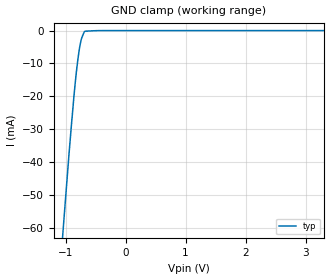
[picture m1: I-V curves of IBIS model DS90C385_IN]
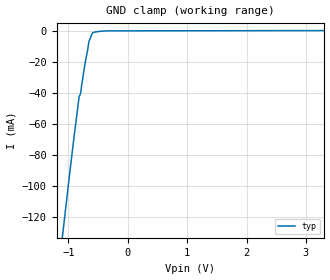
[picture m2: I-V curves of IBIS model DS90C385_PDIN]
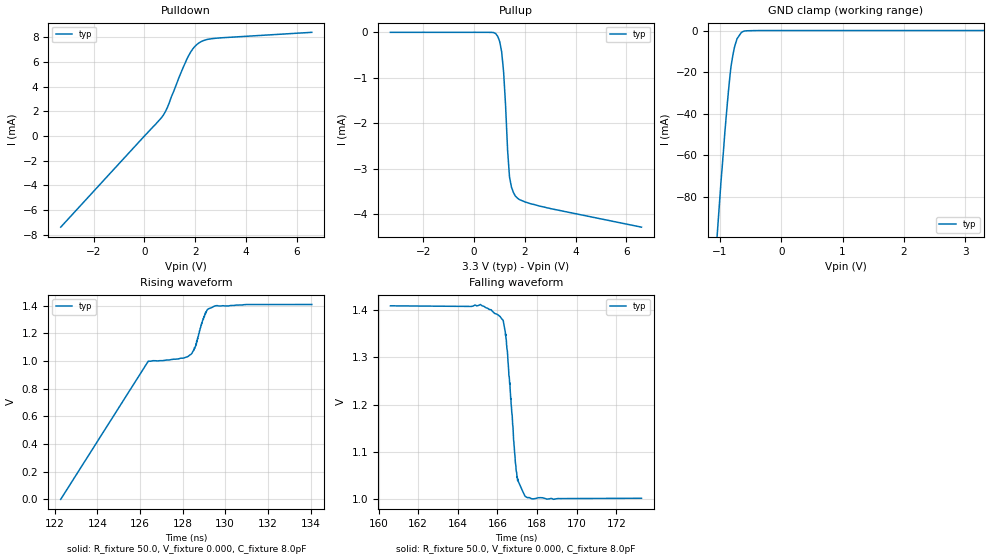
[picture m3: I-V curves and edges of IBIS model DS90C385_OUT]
|   National Semiconductor Corporation
|   Interface Products Group
|   IBIS Model of DS90C385MTD
|   FPD-Link Transmitter
|   56L TSSOP
[IBIS Ver]   2.1
[Comment char]  |_char
[File name]   90c385.ibs
[File Rev]   1.2
[Date]   7/27/00
[Source]   File originated at National Semiconductor Corporation.
   Interface Group/Analog Division. All data based on
   Empirical Measurements(Bench).
[Notes]   File created by DT.
   Revision 1.0: The original model.
   Revision 1.1: Modified driver output pulldown
   and pullup to ensure no double
   counting of clamp current.
   Revision 1.2: Corrected ground and power clamp data.
[Disclaimer]
(C) Copyright National Semiconductor Corporation 2000
   All rights reserved
   National Semiconductor Corporation hereby grants
the user of this IBIS model a non-exclusive, nontransferable
license to use this IBIS model under the following terms.
Before using this IBIS model, the user should read this
license.  If the user does not accept these terms, the
IBIS model should be returned to National within 30 days.
   The user is granted this license only to use the
IBIS model and is not granted rights to sell, load, rent,
lease or license the IBIS model in whole or in part, or in
modified form to anyone other than user. User may modify
the IBIS model to suit its specific applications but rights
to derivative works and such modifications shall belong to
National.
   This IBIS model is provided on an "AS IS" basis and
National makes absolutely no warranty with respect to the
information contained herein. NATIONAL DISCLAIMS AND CUSTOMER
WAIVES ALL WARRANTIES, EXPRESS OR IMPLIED, INCLUDING
WARRANTIES OF MERCHANTABILITY OR FITNESS FOR A PARTICULAR
PURPOSE. The entire risk as to quality and performance is
with the Customer. ACCORDINGLY, IN NO EVENT SHALL THE
COMPANY BE LIABLE FOR ANY DAMAGES, WHETHER IN CONTRACT OR
TORT,INCLUDING ANY LOST PROFITS OR OTHER INCIDENTAL,
CONSEQUENTIAL, EXEMPLARY, OR PUNITIVE DAMAGES ARISING OUT
OF THE USE OR APPLICATION OF THE IBIS model provided in
this package. Further, National reserves the right to make
changes without notice to any product herein to improve
reliability, function, or design. National does not convey
any license under patent rights or any other intellectual
property rights, including those of third parties.
   National is not obligated to provide maintenance or support
for the licensed IBIS model.
Contact National at ATTN:INTERFACE APPLICATIONS/IBIS MODELS.
2900 Semiconductor Drive, M/S A2595, Santa Clara, CA 95052-8090
[Copyright]   Copyright 2000, National Semiconductor, All Rights Reserved
[Component]   DS90C385MTD
[Manufacturer]  National Semiconductor Corp
[Package]
|   typ   min   max
R_pkg   61.4m   NA   NA
L_pkg   1.758nH   NA   NA
C_pkg   0.075pF   NA   NA
[Pin]   signal_name   model_name   R_pin   L_pin   C_pin
1   VCC   POWER   90.0m   3.077n   0.122p
2   TxIN5   DS90C385_IN   90.0m   2.704n   0.107p
3   TxIN6   DS90C385_IN   90.0m   2.405n   0.106p
4   TxIN7   DS90C385_IN   70.0m   2.105n   0.096p
5   GND   GND   70.0m   1.874n   0.080p
6   TxIN8   DS90C385_IN   60.0m   1.619n   0.071p
7   TxIN9   DS90C385_IN   60.0m   1.414n   0.068p
8   TxIN10   DS90C385_IN   60.0m   1.405n   0.068p
9   Vcc   POWER   50.0m   1.407n   0.055p
10   TxIN11   DS90C385_IN   50.0m   1.396n   0.055p
11   TxIN12   DS90C385_IN   50.0m   1.365n   0.055p
12   TxIN13   DS90C385_IN   50.0m   1.318n   0.055p
13   GND   GND   40.0m   1.277n   0.057p
14   TxIN14   DS90C385_IN   30.0m   1.249n   0.061p
15   TxIN15   DS90C385_IN   30.0m   1.249n   0.061p
16   TxIN16   DS90C385_IN   40.0m   1.277n   0.057p
17   R_FB   NC   50.0m   1.318n   0.055p
18   TxIN17   DS90C385_IN   50.0m   1.365n   0.055p
19   TxIN18   DS90C385_IN   50.0m   1.396n   0.055p
20   TxIN19   DS90C385_IN   50.0m   1.407n   0.055p
21   GND   GND   60.0m   1.405n   0.068p
22   TxIN20   DS90C385_IN   60.0m   1.414n   0.068p
23   TxIN21   DS90C385_IN   60.0m   1.619n   0.071p
24   TxIN22   DS90C385_IN   70.0m   1.874n   0.080p
25   TxIN23   DS90C385_IN   70.0m   2.105n   0.096p
26   Vcc   POWER   90.0m   2.405n   0.106p
27   TxIN24   DS90C385_IN   90.0m   2.704n   0.107p
28   TxIN25   DS90C385_IN   90.0m   3.077n   0.122p
29   GND   GND   90.0m   3.077n   0.122p
30   TxIN26   DS90C385_IN   90.0m   2.704n   0.107p
31   TxCLKIN   DS90C385_IN   90.0m   2.405n   0.106p
32   PWRDWN*   DS90C385_PDIN   70.0m   2.105n   0.096p
33   PLLGND   GND   70.0m   1.874n   0.080p
34   PLLVCC   POWER   60.0m   1.619n   0.071p
35   PLLGND   GND   60.0m   1.414n   0.068p
36   LVDSGND   GND   60.0m   1.405n   0.068p
37   TxOUT3+   DS90C385_OUT   50.0m   1.407n   0.055p
38   TxOUT3-   DS90C385_OUT   50.0m   1.396n   0.055p
39   TxCLKOUT   DS90C385_OUT   50.0m   1.365n   0.055p
40   TxCLKOUT   DS90C385_OUT   50.0m   1.318n   0.055p
41   TxOUT2+   DS90C385_OUT   40.0m   1.277n   0.057p
42   TxOUT2-   DS90C385_OUT   30.0m   1.249n   0.061p
43   LVDSGND   GND   30.0m   1.249n   0.061p
44   LVDSVCC   POWER   40.0m   1.277n   0.057p
45   TxOUT1+   DS90C385_OUT   50.0m   1.318n   0.055p
46   TxOUT1-   DS90C385_OUT   50.0m   1.365n   0.055p
47   TxOUT0+   DS90C385_OUT   50.0m   1.396n   0.055p
48   TxOUT0-   DS90C385_OUT   50.0m   1.407n   0.055p
49   LVDSGND   GND   60.0m   1.405n   0.068p
50   TxIN27   DS90C385_IN   60.0m   1.414n   0.068p
51   TxIN0   DS90C385_IN   60.0m   1.619n   0.071p
52   TxIN1   DS90C385_IN   70.0m   1.874n   0.080p
53   GND   GND   70.0m   2.105n   0.096p
54   TxIN2   DS90C385_IN   90.0m   2.405n   0.106p
55   TxIN3   DS90C385_IN   90.0m   2.704n   0.107p
56   TxIN4   DS90C385_IN   90.0m   3.077n   0.122p
[Diff_pin]   inv_pin   vdiff   tdelay_typ   tdelay_min   tdelay_max
| The '+' pin is Diff_pin and the '-' pin is the inv_pin
37   38   0.1   0   0   0
39   40   0.1   0   0   0
41   42   0.1   0   0   0
45   46   0.1   0   0   0
47   48   0.1   0   0   0
| Models and submodels in the file (3): DS90C385_IN (Input), DS90C385_PDIN (Input), DS90C385_OUT (3-state)
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|   Driver Input  MODEL
[Model]   DS90C385_IN
Model_type   Input
|Signals   TxIN0 ~ TxIN27
Vinh = 2.0
Vinl = 0.8
|   typ   min   max
C_comp   5.910pF   NA   NA
|   typ   min   max
[Temperature Range]   25.0   NA   NA
[Voltage range]   3.3V   3.0V   3.6V
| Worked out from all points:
|   GND clamp passes 1 mA (typ) near -0.70 V on its own axis
[Power_clamp]
| Note that the[POWER_clamp]voltage table is referenced to Vcc
| and is calculated using Vtable=Vcc - Vmeasured.
|Voltage   I(typ)   I(min)   I(max)
-3V       0A         NA         NA
3V        0A         NA         NA
[GND_clamp]
|Voltage   I(typ)   I(min)   I(max)
-3.3V     -594.1mA   NA         NA
-1.001V   -51.39mA   NA         NA
-941.2mV  -37.29mA   NA         NA
-899.9mV  -28.27mA   NA         NA
-859.6mV  -19.87mA   NA         NA
-818.3mV  -12.37mA   NA         NA
-776.9mV  -6.424mA   NA         NA
-756.3mV  -4.202mA   NA         NA
-736.1mV  -2.573mA   NA         NA
-717mV    -1.615mA   NA         NA
-675.2mV  -194.8uA   NA         NA
3.3V      524nA      NA         NA
|   Driver PWRDWN* Input  MODEL
[Model]   DS90C385_PDIN
Model_type   Input
|Signals   PWRDWN*
Vinh = 2.0
Vinl = 0.8
|   typ   min   max
C_comp   5.843pF   NA   NA
|   typ   min   max
[Temperature Range]   25.0   NA   NA
[Voltage range]   3.3V   3.0V   3.6V
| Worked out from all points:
|   GND clamp passes 1 mA (typ) near -0.57 V on its own axis
[Power_clamp]
| Note that the[POWER_clamp]voltage table is referenced to Vcc
| and is calculated using Vtable=Vcc - Vmeasured.
|Voltage   I(typ)   I(min)   I(max)
-3V       0A         NA         NA
3V        0A         NA         NA
[GND_clamp]
|Voltage   I(typ)   I(min)   I(max)
-3.3V     -863.2mA   NA         NA
-999.7mV  -98.78mA   NA         NA
-918.6mV  -72.42mA   NA         NA
-819.7mV  -42.41mA   NA         NA
-796.1mV  -40.44mA   NA         NA
-776.9mV  -35.09mA   NA         NA
-735.6mV  -24.85mA   NA         NA
-674.7mV  -11.91mA   NA         NA
-655mV    -6.957mA   NA         NA
-592.5mV  -1.248mA   NA         NA
-306.8mV  -9.428uA   NA         NA
3.3V      172.6uA    NA         NA
|   Driver Output  MODEL
[Model]   DS90C385_OUT
Model_type   3-state
| Signals   TxOUT0 ~ TxOUT3; TxCLKOUT
Vmeas = 1.2V   |This is 0.0v differential on output
Cref = 5pF   |Timing specification test load capacitance value
Rref = 50   |Note: 100 Ohm between the two driver outputs
Vref = 1.2   |Timing specification test load voltage; GND
| variable   typ   min   max
C_comp   6.704pF   NA   NA
|   typ   min   max
[Temperature Range]   25.0   NA   NA
[Voltage range]   3.3V   3.0V   3.6V
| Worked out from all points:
|   slope of the pulldown table from 0 to 0.495 V, typ, clamps not added: 459 ohm
|   GND clamp passes 1 mA (typ) near -0.65 V on its own axis
|   rising waveform, R_fixture 50.0, V_fixture 0.000, C_fixture 8.0pF: 20-80 % time 5.21ns typ, NA min, NA max; typ from 0 V to 1.41 V
|   falling waveform, R_fixture 50.0, V_fixture 0.000, C_fixture 8.0pF: 20-80 % time 438ps typ, NA min, NA max; typ from 1.41 V to 1 V
[Pulldown]
| Voltage   I(typ)   I(min)   I(max)
-3.3V     -7.392mA   NA         NA
667.8mV   1.466mA    NA         NA
748mV     1.688mA    NA         NA
907.8mV   2.312mA    NA         NA
1.372V    4.782mA    NA         NA
1.681V    6.257mA    NA         NA
1.909V    7.054mA    NA         NA
2.136V    7.516mA    NA         NA
2.442V    7.802mA    NA         NA
2.749V    7.903mA    NA         NA
6.6V      8.398mA    NA         NA
[Pullup]
| Note that the[Pullup]voltage table is referenced to Vcc
| and is calculated using Vtable=Vcc - Vmeasured.
|Voltage   I(typ)   I(min)   I(max)
-3.3V     -524nA     NA         NA
854.5mV   -29.33uA   NA         NA
1.009V    -203.2uA   NA         NA
1.087V    -429.5uA   NA         NA
1.164V    -876.3uA   NA         NA
1.242V    -1.62mA    NA         NA
1.32V     -2.587mA   NA         NA
1.396V    -3.187mA   NA         NA
1.474V    -3.411mA   NA         NA
1.629V    -3.606mA   NA         NA
2.559V    -3.822mA   NA         NA
6.6V      -4.289mA   NA         NA
[GND_clamp]
| Outputs in Tri-state.
| Voltage   I(typ)   I(min)   I(max)
-3.3V     -1.034A    NA         NA
-1.001V   -81.02mA   NA         NA
-983mV    -73.48mA   NA         NA
-921.5mV  -50.22mA   NA         NA
-900.9mV  -42.95mA   NA         NA
-859.6mV  -29.11mA   NA         NA
-819.2mV  -17.54mA   NA         NA
-767.2mV  -8.785mA   NA         NA
-719.4mV  -3.945mA   NA         NA
-634.3mV  -657.5uA   NA         NA
-347.7mV  -11.87uA   NA         NA
3.3V      524nA      NA         NA
[POWER_clamp]
| Note that the[POWER_clamp]voltage table is referenced to Vcc
| and is calculated using Vtable=Vcc - Vmeasured.
| Outputs in Tri-state.
|Voltage   I(typ)   I(min)   I(max)
-3V       0A         NA         NA
3V        0A         NA         NA
[Ramp]
| Note: Ramp rate measured on single-ended Driver Output.
|   typ   min   max
dV/dt_r   204.0m/446.03p   NA   NA
dV/dt_f   205.5m/372.29p   NA   NA
R_load = 100Ohm | Note: This 100 Ohm is across the two driver output
[Rising Waveform]
R_fixture = 50.0
V_fixture = 0.000
C_fixture = 8.0pF
|Time   V(typ)   V(min)  V(max)
122.3ns   0V         NA         NA
126.4ns   999.4mV    NA         NA
128ns     1.021V     NA         NA
128.4ns   1.048V     NA         NA
128.6ns   1.118V     NA         NA
128.7ns   1.145V     NA         NA
128.9ns   1.259V     NA         NA
129.2ns   1.372V     NA         NA
129.6ns   1.401V     NA         NA
134.1ns   1.409V     NA         NA
[Falling Waveform]
R_fixture = 50.0
V_fixture = 0.000
C_fixture = 8.0pF
|Time   V(typ)   V(min)  V(max)
160.6ns   1.41V      NA         NA
165.1ns   1.412V     NA         NA
166.3ns   1.379V     NA         NA
166.4ns   1.349V     NA         NA
166.5ns   1.314V     NA         NA
166.8ns   1.122V     NA         NA
166.9ns   1.059V     NA         NA
167ns     1.039V     NA         NA
167.4ns   1.005V     NA         NA
173.3ns   1.001V     NA         NA
